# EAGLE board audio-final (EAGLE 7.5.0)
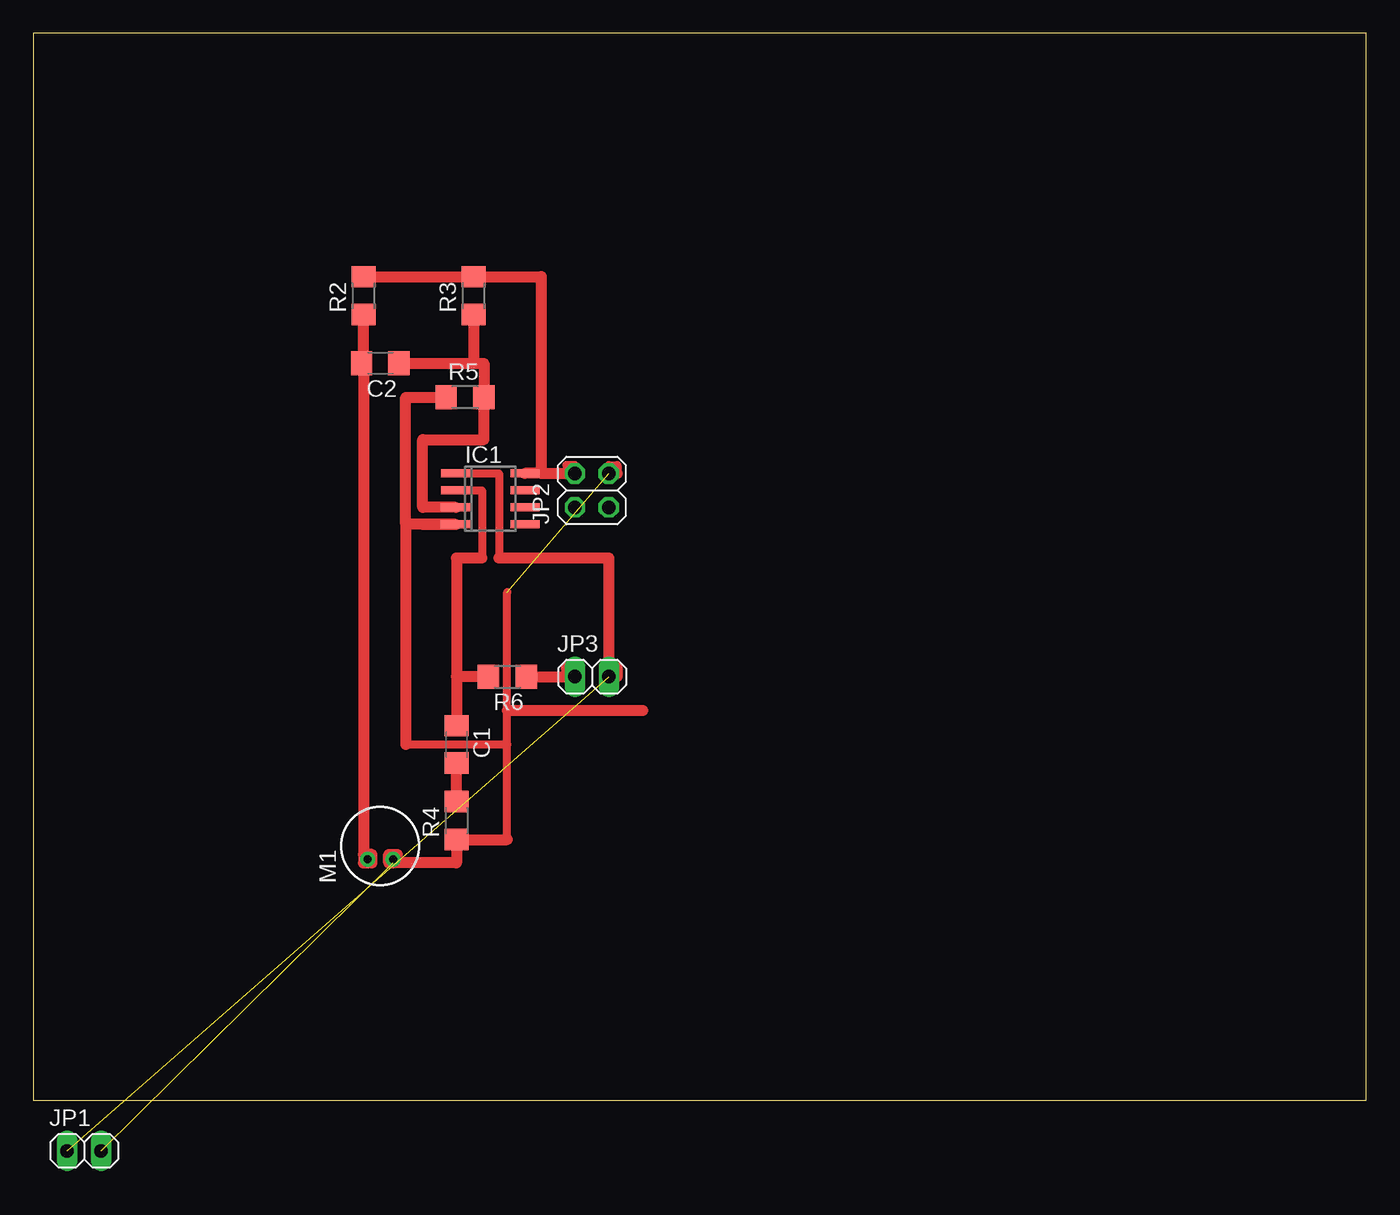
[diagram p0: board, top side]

Size 100 x 80 mm. Coordinates in mm from the lower left corner, seen from the top.
Outline: 0,0 100,0 100,80 0,80 0,0
Copper layers (1*16): Top 0.035mm / dielectric 1.5mm / Bottom 0.035mm
Design rules "default": minimum track width 10mil, minimum drill 24mil, track to track 8mil, track to pad 8mil, pad to pad 8mil, via to via 8mil, smd to smd 8mil, copper to edge 40mil, drill to drill 8mil, minimum pad ring 10mil, minimum via ring 8mil, stop-mask expansion 4mil, vias tented up to drill 0mil, thermal gap 10mil

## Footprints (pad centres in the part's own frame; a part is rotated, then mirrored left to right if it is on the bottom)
C1206 = smd 1.6 x 1.8: 1 -1.4,0; 2 1.4,0
SO08 = smd 0.6 x 2.2: 1 -1.905,-2.6; 2 -0.635,-2.6; 3 0.635,-2.6; 4 1.905,-2.6; 5 1.905,2.6; 6 0.635,2.6; 7 -0.635,2.6; 8 -1.905,2.6
1X02 = drill 1.016 long: 1 -1.27,0; 2 1.27,0
2X02 = drill 1.016 octagon: 1 -1.27,-1.27; 2 -1.27,1.27; 3 1.27,-1.27; 4 1.27,1.27
WM-62PC/62PK = drill 0.6 pad 1: 1 -1,0.95; 2 -1,-0.95
R1206 = smd 1.6 x 1.803: 1 -1.422,0; 2 1.422,0

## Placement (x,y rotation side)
C1  1uF  [C1206]  31.75,26.67 270 top
C2  1uF  [C1206]  26.04,55.24 180 top
IC1  TL072D  [SO08]  34.29,45.09 270 top
JP1  [1X02]  not placed on the board
JP2  5V  [2X02]  41.91,45.72 90 top
JP3  Potentiom  [1X02]  41.91,31.75 0 top
M1  ELECTRET_MICROPHON-WM-62PC/62PK  [WM-62PC/62PK]  26.04,19.05 90 top
R2  10K  [R1206]  24.77,60.33 90 top
R3  100k  [R1206]  33.02,60.33 90 top
R4  2K  [R1206]  31.75,20.95 90 top
R5  100k  [R1206]  32.38,52.7 0 top
R6  0  [R1206]  35.56,31.75 180 top

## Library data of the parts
C1 C2 = rcl
IC1 = linear
JP1-JP3 = pinhead
M1 = microphon
R2-R6 = resistor

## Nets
AGND: IC1.4 JP1.2 JP2.3 M1.2 R4.1 R5.1
N$1: JP3.1 R6.1
N$2: IC1.8 JP2.4 R2.2 R3.2
N$3: IC1.1 JP1.1 JP3.2
N$4: C1.1 IC1.2 R6.2
N$6: C2.1 IC1.3 R3.1 R5.2
N$7: C2.2 M1.1 R2.1
N$9: C1.2 R4.2

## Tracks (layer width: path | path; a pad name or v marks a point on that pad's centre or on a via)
AGND  (2 unrouted)
  Top 0.61: JP2.3 43.18,47.62 43.81,47.62 43.81,46.99 | 35.56,19.53 35.56,26.67 | 35.56,26.67 35.56,29.21 35.56,38.1 | 27.94,26.67 35.56,26.67
  Top 0.813: 35.56,19.53 R4.1 31.75,17.78 26.98,17.78 M1.2 | 29.21,43.18 IC1.4 27.94,43.18 | 27.94,43.18 27.94,52.7 R5.1 | JP2.3 43.81,46.99 | 27.94,43.18 27.94,26.67 | 45.72,29.21 35.56,29.21
N$1
  Top 0.813: R6.1 40.01,31.75 | 40.01,31.75 JP3.1 40.64,32.38 40.01,32.38 40.01,31.75
N$2
  Top 0.61: JP2.4 40.64,47.62 40.01,47.62 40.01,46.99
  Top 0.813: 38.1,46.99 IC1.8 | R2.2 R3.2 38.1,61.75 38.1,46.99 | 38.1,46.99 40.01,46.99 JP2.4
N$3  (1 unrouted)
  Top 0.61: IC1.1 34.92,46.99 34.92,40.64
  Top 0.813: 34.92,40.64 43.18,40.64 43.18,38.1 43.18,32.38 | 43.18,32.38 JP3.2 43.81,31.75 43.81,32.38 43.18,32.38
N$4
  Top 0.61: IC1.2 33.66,45.72 33.66,40.64
  Top 0.813: 31.75,31.75 C1.1 | 33.66,40.64 31.75,40.64 31.75,31.75 | R6.2 31.75,31.75
N$6
  Top 0.813: IC1.3 29.21,44.45 29.21,49.53 33.81,49.53 R5.2 33.81,55.24 33.02,55.24 | C2.1 33.02,55.24 | R3.1 33.02,55.24
N$7
  Top 0.813: 25.4,17.78 25.4,18.41 24.77,18.41 | 24.77,55.24 24.77,18.41 | 24.77,18.41 24.77,17.78 25.09,17.78 M1.1 | C2.2 24.77,55.24 | 24.77,55.24 R2.1
N$8
  Top 0.813: 26.67,17.78 26.67,18.41 27.3,18.41
N$9
  Top 0.813: R4.2 C1.2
